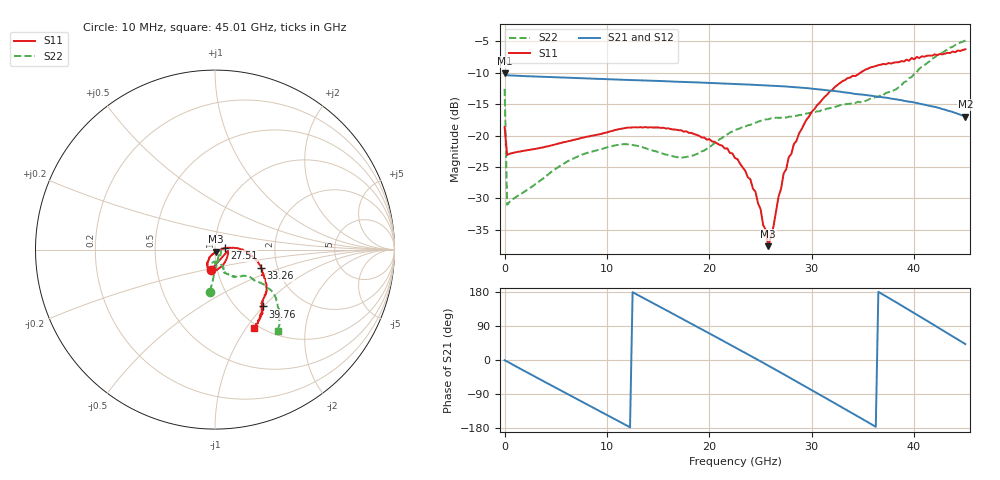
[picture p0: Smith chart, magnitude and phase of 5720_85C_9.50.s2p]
! Device:  ADRF5720
! Description: 0.5dB LSB GaAs MMIC 6-bit Digital Attenuator
! Frequency:  0.000009 -  40 GHz
! Ports:
!	RF1	= Port 1
!	RF2	= Port 2
! Vdd:  3.3 Volt
! Vss:  -3.3 Volt
! Control:  0/3.3 Volt
! State:  9.50 dB attenuation
! Data:  The device was measured using G-S-G Probes on a matrix board.
!  Data was collected using an calibrated 4 port network analyzer.
!  The reference plane for this measurement is at the launchers.
! Note:  Analog Devices supplies this data as a sample of measured data
!  for this product.  Your particular data for this product may vary.
!  Data was taken at 85 degrees C.
!  Analog Devices reserves the right to change this data at anytime.
# GHZ S DB R 45.0
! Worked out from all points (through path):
!   181 points, 10 MHz to 45.01 GHz, reference 45 ohm
!   highest |S21| = -10.11 dB at 10 MHz (marker M1); lowest = -17.0 dB at 45.01 GHz (marker M2)
!   group delay of S21, straight-line fit = 41.5 ps
!   lowest |S11| = -37.6 dB at 25.76 GHz (marker M3), VSWR 1.03, Z = 45.4 - j1.12 ohm
!   |S11| at or under -10 dB: start of sweep to 34.75 GHz
!   |S22| runs from -31.0 to -4.8 dB; largest |S21 - S12| = 0.0014
!   S11 on the Smith chart (normalised r, x): 10 MHz: 0.93, -0.22; 27.51 GHz: 1.11, +0.02; 33.26 GHz: 1.64, -0.37; 39.76 GHz: 1.30, -1.00; 45.01 GHz: 0.95, -1.09
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0.01  -18.62 -101.8  -10.11 -0.8  -10.10 -0.8  -12.56 -96.7
0.26  -23.09 -8.1  -10.40 -4.0  -10.39 -4.0  -31.02 -16.8
4.26  -21.71 -38.9  -10.67 -62.5  -10.65 -62.5  -26.20 -56.3
7.76  -20.32 -62.7  -10.88 -112.9  -10.86 -112.8  -22.93 -79.2
11.51  -18.87 -85.0  -11.11 -166.8  -11.10 -166.7  -21.39 -96.3
15.26  -18.78 -103.7  -11.31 139.2  -11.30 139.3  -22.77 -100.5
19.01  -20.05 -115.7  -11.55 84.8  -11.53 84.9  -22.79 -75.1
22.76  -23.77 -121.4  -11.80 29.8  -11.79 30.0  -18.99 -65.9
24.51  -28.95 -119.1  -11.93 3.9  -11.91 4.1  -17.95 -68.0
25.51  -35.01 -83.2  -12.00 -11.0  -11.98 -10.8  -17.41 -68.9
25.76  -37.62 -69.5  -12.02 -14.8  -12.00 -14.6  -17.41 -68.3
26.26  -34.54 -17.4  -12.06 -22.4  -12.04 -22.1  -17.24 -68.0
27.26  -26.02 6.0  -12.16 -37.5  -12.15 -37.3  -17.11 -67.3
27.51  -25.37 9.9  -12.19 -41.3  -12.17 -41.1  -17.13 -66.4
28.26  -21.34 7.2  -12.28 -52.8  -12.27 -52.5  -16.86 -66.4
30.26  -15.80 -2.9  -12.57 -83.4  -12.55 -83.1  -16.36 -62.7
33.26  -11.17 -21.9  -13.13 -129.8  -13.11 -129.5  -15.02 -56.6
35.51  -9.33 -33.5  -13.59 -164.6  -13.57 -164.2  -14.30 -51.7
37.76  -8.53 -42.4  -14.11 159.9  -14.09 160.3  -12.88 -40.6
39.76  -7.64 -49.8  -14.64 127.8  -14.62 128.2  -10.68 -37.6
42.26  -7.17 -54.5  -15.53 87.0  -15.50 87.4  -7.21 -38.6
45.01  -6.26 -63.4  -16.97 41.9  -16.94 42.3  -4.85 -52.0
